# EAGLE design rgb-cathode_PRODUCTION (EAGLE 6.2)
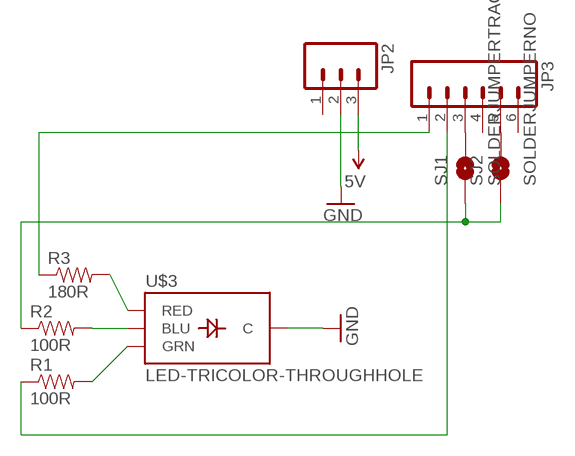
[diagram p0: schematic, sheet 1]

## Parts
JP2  M03PTH  [1X03]
JP3  M06SIP  [1X06]
R1  100R  RESISTORAXIAL-0.3  [AXIAL-0.3]
R2  100R  RESISTORAXIAL-0.3  [AXIAL-0.3]
R3  180R  RESISTORAXIAL-0.3  [AXIAL-0.3]
SJ1  SOLDERJUMPERTRACE  [SJ_2S-TRACE]
SJ2  SOLDERJUMPERNO  [SJ_2S-NO]
U$3  LED-TRICOLOR-THROUGHHOLE  [LED-TRICOLOR-THROUGHHOLE]

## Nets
5V: JP2.3
GND: JP2.2 U$3.GND(C)
N$1: R3.P$2 U$3.RED
N$2: R2.P$2 U$3.BLU
N$3: R1.P$2 U$3.GRN
N$4: JP3.1 R3.P$1
N$5: R2.P$1 SJ1.1 SJ2.1
N$6: JP3.2 R1.P$1
N$7: JP3.3 SJ1.2
N$8: JP3.5 SJ2.2
Unconnected: JP2.1 JP3.4 JP3.6

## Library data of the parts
JP2 = SparkFun:M03: Header 3 Standard 3-pin 0.1" header. Use with straight break away headers (SKU : PRT-00116), right angle break away headers (PRT-00553), swiss pins (PRT-00743), machine pins (PRT-00117), and female headers (PRT-00115). Molex polarized connector foot print use with SKU : PRT-08232 with associated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
JP3 = SparkFun:M06: Header 6 Standard 6-pin 0.1" header. Use with straight break away headers (SKU : PRT-00116), right angle break away headers (PRT-00553), swiss pins (PRT-00743), machine pins (PRT-00117), and female headers (PRT-00115). Molex polarized connector foot print use with SKU : PRT-08094 with associated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
R1-R3 = SparkFun:RESISTOR: Resistor
SJ1 SJ2 = SparkFun:SOLDERJUMPER: Solder Jumper
U$3 = SparkFun:LED-TRICOLOR-THROUGHHOLE

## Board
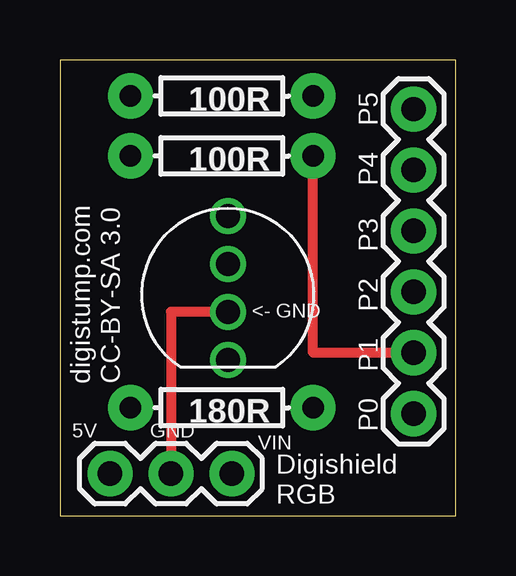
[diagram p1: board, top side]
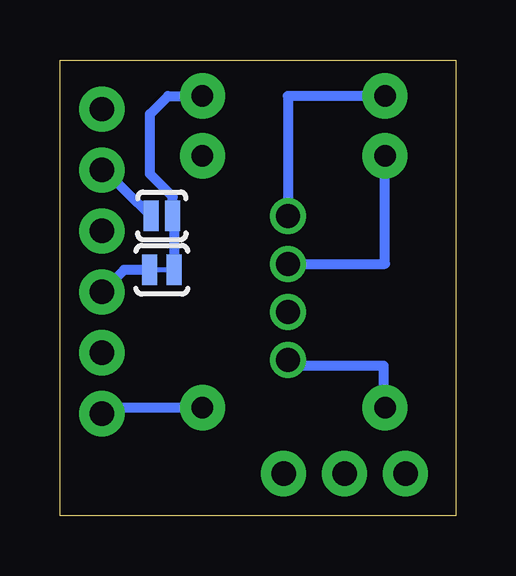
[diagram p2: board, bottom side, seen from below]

Size 16.5 x 19 mm. Coordinates in mm from the lower left corner, seen from the top.
Outline: 0,19 0,0 16.5,0 16.5,19 0,19
Copper layers (1*16): Top 0.0356mm / dielectric 1.5011mm / Bottom 0.0356mm
Design rules: minimum track width 12mil, minimum drill 13mil, track to track 12mil, track to pad 12mil, pad to pad 12mil, via to via 12mil, smd to smd 8mil, copper to edge 15mil, drill to drill 12mil, minimum pad ring 7mil, minimum via ring 7mil, stop-mask expansion 4mil, vias tented up to drill 0mil, thermal gap 10mil

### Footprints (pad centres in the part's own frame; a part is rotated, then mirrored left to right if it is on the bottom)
1X03 = drill 1.016 pad 1.88: 1 0,0; 2 2.54,0; 3 5.08,0
1X06 = drill 1.016 pad 1.88: 1 0,0; 2 2.54,0; 3 5.08,0; 4 7.62,0; 5 10.16,0; 6 12.7,0
AXIAL-0.3 = drill 0.9 pad 1.88: P$1 -3.81,0; P$2 3.81,0
SJ_2S-TRACE = smd 0.635 x 1.27: 1 -0.508,0; 2 0.508,0
SJ_2S-NO = smd 0.635 x 1.27: 1 -0.45,0; 2 0.45,0
LED-TRICOLOR-THROUGHHOLE = drill 1: BLU 3,0; GND -1,0; GRN 1,0; RED -3,0

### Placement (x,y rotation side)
JP2  7.17,1.75 180 top
JP3  14.75,4.25 90 top
R1  6.75,15 180 top
R2  6.75,17.5 180 top
R3  6.75,4.5 180 top
SJ1  12.25,10.25 180 bottom
SJ2  12.25,12.5 180 bottom
U$3  7,9.5 90 top

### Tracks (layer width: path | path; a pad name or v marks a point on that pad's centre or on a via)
GND
  Top 0.406: U$3.GND 4.63,8.5 JP2.2
N$1
  Bottom 0.406: R3.P$2 3,4.5 3,6.25 7,6.25 U$3.RED
N$2
  Bottom 0.406: R2.P$2 7,17.5 U$3.BLU
N$3
  Bottom 0.406: U$3.GRN 2.94,10.5 R1.P$2
N$4
  Bottom 0.406: R3.P$1 14.75,4.5 JP3.1
N$5
  Bottom 0.406: R2.P$1 12,17.5 12.75,16.75 12.75,14.25 11.8,13.3 SJ2.1 11.74,12.5 SJ1.1
N$6
  Top 0.406: JP3.2 10.56,6.79 R1.P$1
N$7
  Bottom 0.406: SJ1.2 13.83,10.25 JP3.3
N$8
  Bottom 0.406: SJ2.2 14.75,14.5 JP3.5

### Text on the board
tPlace: P5 | P4 | P3 | <- | GND | P2 | digistump.com | CC-BY-SA 3.0 | P1 | P0 | 5V | GND | VIN | Digishield | RGB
